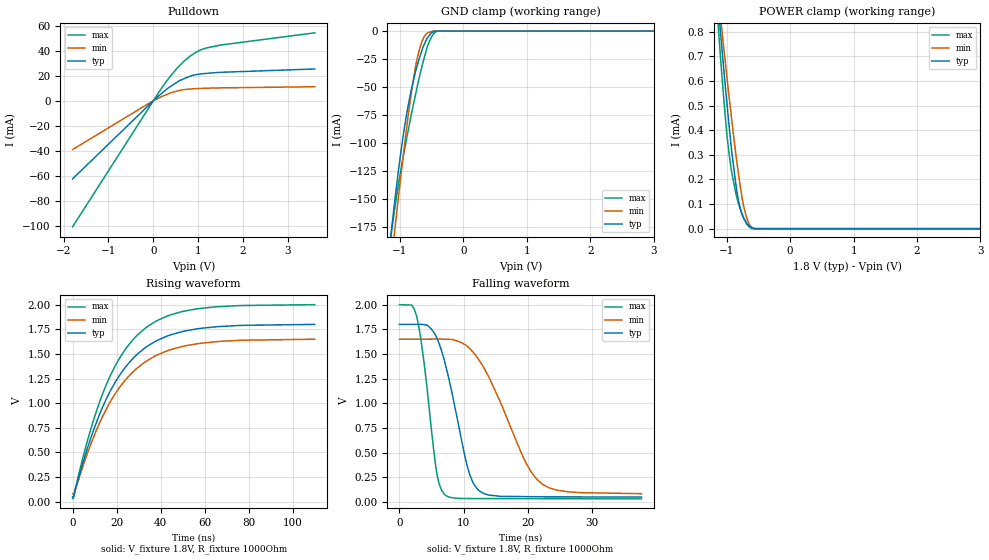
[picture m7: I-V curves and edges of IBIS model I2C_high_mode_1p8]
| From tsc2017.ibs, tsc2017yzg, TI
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|   i2c_high_mode_1p8 Model
[Model]   I2C_high_mode_1p8
Model_type   I/O_open_drain
Polarity   Non-Inverting
Enable   Active-Low
Vinl = 0.54
Vinh = 1.26
Vmeas = 0.9
Vref = 1.8
Cref = 100pF
Rref = 1000
|   typ   min   max
|   (nom PVT)   (Fast PVT)   (slow PVT)
|Average
C_comp   1.636e-11   1.570e-11   1.694e-11
|ON state : BUFFER OUTPUT TURNED LOW
|C_comp   4.183e-11   3.468e-11   4.200e-11
|OFF state: BUFFER in HIGH IMPEDANCE
|C_comp   1.636e-11   1.570e-11   1.694e-11
|C_comp from frequency method(F=3.4MHz)
| Where nom  PVT is Nominal Process, 1.8V, 25C
|   Fast PVT is Strong Process,  2V, -40C
|   Slow PVT is Weak Process,   1.65V, 85C
[Model Spec]
Vinl   0.54   0.495   0.6
Vinh   1.26   1.155   1.4
[Voltage Range]   1.8   1.65   2
|Ambient Temperature   25   85   -40
|Junction Temperature
[Temperature Range]   25   85   -40
[Pullup Reference]   1.8   1.65   2
[Pulldown Reference]   0   0   0
[Power Clamp Reference]   1.8   1.65   2
[GND Clamp Reference]   0   0   0
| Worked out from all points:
|   slope of the pulldown table from 0 to 0.27 V, typ, clamps not added: 32 ohm
|   GND clamp passes 1 mA (typ) near -0.48 V on its own axis
|   POWER clamp passes 1 mA (typ) near -1.17 V on its own axis
|   falling waveform, V_fixture 1.8V, R_fixture 1000Ohm: 20-80 % time 3.49ns typ, 6.37ns min, 2.09ns max; typ from 1.8 V to 0.051 V
|   rising waveform, V_fixture 1.8V, R_fixture 1000Ohm: 20-80 % time 22.5ns typ, 23.1ns min, 21.6ns max; typ from 0.051 V to 1.8 V
[Pulldown]
|   Voltage   I(typ)   I(min)   I(max)
-1.8V     -62.32mA   -38.9mA    -100.6mA
-102.2mV  -3.57mA    -2.096mA   -5.745mA
142mV     4.543mA    2.624mA    7.89mA
428mV     12.49mA    6.872mA    21.76mA
577.8mV   15.99mA    8.178mA    27.78mA
828mV     19.82mA    9.449mA    35.86mA
1.064V    21.55mA    9.913mA    40.79mA
1.498V    22.77mA    10.34mA    44.52mA
3.6V      25.44mA    11.26mA    54.29mA
[GND Clamp]
|   Voltage   I(typ)   I(min)   I(max)
-1.8V     -554.1mA   -567.1mA   -560.8mA
-1.15V    -186.5mA   -213.7mA   -186.5mA
-1.085V   -153.9mA   -180mA     -160.5mA
-1.076V   -149.4mA   -175.2mA   -156.7mA
-925.2mV  -84.72mA   -101.1mA   -105.1mA
-856.2mV  -62.68mA   -69.86mA   -85.05mA
-757.2mV  -37.1mA    -32.55mA   -57.67mA
-656.5mV  -18.02mA   -9.927mA   -32.4mA
-570.7mV  -6.514mA   -1.785mA   -14.58mA
-468mV    -361.9uA   0A         -2.378mA
-388mV    0A         0A         0A
3.6V      0A         0A         0A
[POWER Clamp]
|   Voltage   I(typ)   I(min)   I(max)
-1.8V     2.967mA    2.622mA    3.431mA
-1.13V    891.2uA    937uA      808.9uA
-1.106V   819.6uA    877.5uA    720.8uA
-1.064V   696.2uA    775.3uA    582.1uA
-998mV    511.7uA    618uA      382.4uA
-926mV    325.3uA    452.4uA    236.2uA
-862.2mV  192uA      313.9uA    150.3uA
-806.4mV  103uA      206.5uA    94.43uA
-727.5mV  40.37uA    84.06uA    40.29uA
-638mV    9.164uA    15.43uA    4.889uA
-570.7mV  1.367uA    0A         0A
3.6V      0A         0A         0A
[Ramp]
R_load = 1000
|   typ   min   max
dV/dt_r   1.04872/2.24538e-08   0.940871/2.30607e-08   1.17888/2.15397e-08
dV/dt_f   1.04936/3.49232e-09   0.941607/6.37432e-09   1.1794/2.09005e-09
[Falling Waveform]
V_fixture = 1.8V
V_fixture_min = 1.65V
V_fixture_max = 2V
R_fixture = 1000Ohm
|   Time   V(typ)   V(min)   V(max)
0s        1.8V       1.65V      2V
2.725ns   1.801V     1.65V      1.873V
3.85ns    1.798V     1.651V     1.411V
5.75ns    1.675V     1.651V     325.6mV
7.125ns   1.406V     1.65V      73mV
10.6ns    358.9mV    1.578V     36.17mV
12.45ns   114.7mV    1.435V     35.62mV
19.83ns   55.11mV    384.9mV    34.64mV
22.2ns    53.72mV    184.9mV    34.51mV
37.73ns   51.27mV    84.78mV    34.34mV
[Rising Waveform]
V_fixture = 1.8V
V_fixture_min = 1.65V
V_fixture_max = 2V
R_fixture = 1000Ohm
|   Time   V(typ)   V(min)   V(max)
0s        51.07mV    80.65mV    34.34mV
300ps     49.84mV    80.67mV    31.38mV
825ps     85.58mV    85.75mV    90.97mV
8.3ns     647.1mV    584.2mV    737.8mV
15.27ns   1.04V      938.3mV    1.186V
23.3ns    1.344V     1.217V     1.524V
32.43ns   1.553V     1.409V     1.75V
42.85ns   1.679V     1.53V      1.882V
56.42ns   1.753V     1.602V     1.956V
110ns     1.799V     1.649V     1.999V
